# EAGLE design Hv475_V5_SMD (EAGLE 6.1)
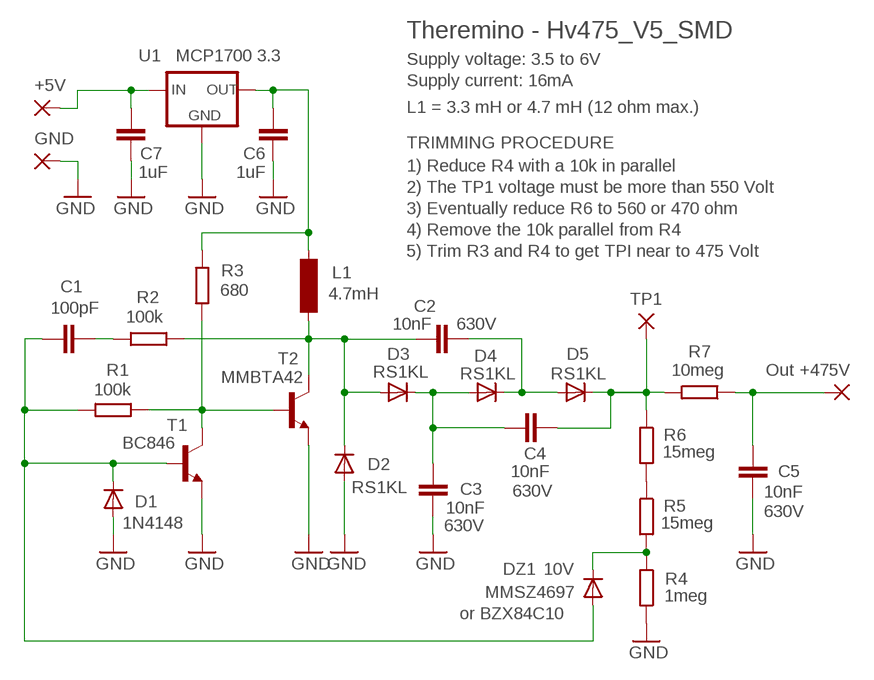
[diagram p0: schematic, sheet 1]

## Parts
+5V  WIREPADSMD2,54-3,81  [SMD2,54-3,81]
+475V  WIREPADSMD1,90-2,54  [SMD1,90-2,54]
C1  100pF  C-EUC0805  [C0805]
C2  10nF  C-EUC1206  [C1206]
C3  10nF  C-EUC1206  [C1206]
C4  10nF  C-EUC1206  [C1206]
C5  10nF  C-EUC1206  [C1206]
C6  1uF  C-EUC0805  [C0805]
C7  1uF  C-EUC0805  [C0805]
D1  1N4148  DIODE-SOD123-LARGE  [SOD123-LARGE]
D2  RS1KL  DIODE-SOD123-LARGE  [SOD123-LARGE]
D3  RS1KL  DIODE-SOD123-LARGE  [SOD123-LARGE]
D4  RS1KL  DIODE-SOD123-LARGE  [SOD123-LARGE]
D5  RS1KL  DIODE-SOD123-LARGE  [SOD123-LARGE]
DZ1  MMSZ4697  DIODE-SOD123-LARGE  [SOD123-LARGE]
GND  WIREPADSMD2,54-3,81  [SMD2,54-3,81]
L1  4.7mH  INDUCTOR_4.7MH472KU  [MSD75]
R1  100k  R-EU_R0805  [R0805]
R2  100k  R-EU_R0805  [R0805]
R3  680  R-EU_R1206_L  [R1206_L]
R4  1meg  R-EU_R0805  [R0805]
R5  15meg  R-EU_R1206  [R1206]
R6  15meg  R-EU_R1206  [R1206]
R7  10meg  R-EU_R1206  [R1206]
T1  BC846  BC846L  [SOT23_L@1]
T2  MMBTA42  -NPN-BC846  [SOT23_L@1]
TP1  TEST  WIREPADSMD1,27-1,27  [SMD1,27-1,27]
U1  MCP1700 3.3  MCP1700SOT23  [SOT23]

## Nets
+5V: C6.1 L1.1 R3.2 U1.2(OUT)
GND: C3.1 C5.1 C6.2 C7.2 D1.A D2.A GND.1(P) R4.1 T1.2(E) T2.2(E) U1.1(GND)
N$1: DZ1.C R4.2 R5.2
N$2: C1.2 R2.2
N$3: R5.1 R6.2
N$4: C1.1 D1.C DZ1.A R1.2 T1.1(B)
N$5: C4.2 D5.C R6.1 R7.2 TP1.1(P)
N$6: C2.1 D2.C D3.A L1.2 R2.1 T2.3(C)
N$7: +5V.1(P) C7.1 U1.3(IN)
N$11: C3.2 C4.1 D3.C D4.A
N$15: +475V.1(P) C5.2 R7.1
N$17: C2.2 D4.C D5.A
N$26: R1.1 R3.1 T1.3(C) T2.1(B)

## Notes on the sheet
- Theremino - Hv475_V5_SMD
- Supply voltage: 3.5 to 6V
- Supply current: 16mA
- L1 = 3.3 mH or 4.7 mH (12 ohm max.)
- TRIMMING PROCEDURE
- 1) Reduce R4 with a 10k in parallel
- 2) The TP1 voltage must be more than 550 Volt
- 3) Eventually reduce R6 to 560 or 470 ohm
- 4) Remove the 10k parallel from R4
- 5) Trim R3 and R4 to get TPI near to 475 Volt
- Out +475V

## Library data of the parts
+5V +475V GND TP1 = 00-LIVIO:WIREPAD: Wire PAD connect wire on PCB
C1 C6 C7 = 00-LIVIO:C-EU: CAPACITOR, European symbol
C2-C5 = 00-LIVIO:C-EU: CAPACITOR, European symbol; VOLTAGE: 630V
D1-D5 = 00-LIVIO:DIODE-: DIODE
DZ1 = 00-LIVIO:DIODE-: DIODE; EQUIVALENT: or BZX84C10; VZ: 10V
L1 = 00-LIVIO:INDUCTOR_4.7MH: INDUCTOR
R1-R7 = 00-LIVIO:R-EU_: RESISTOR, European symbol
T1 = 00-LIVIO:BC846
T2 = 00-LIVIO:*-NPN-: NPN Transistror
U1 = 00-LIVIO:MCP1700: Linear regulator Quescient courrent 1.8uA Input 2.3v to 6v Output 1.2v 1.8v 2.5v 3.0v 3.3v 5.0v

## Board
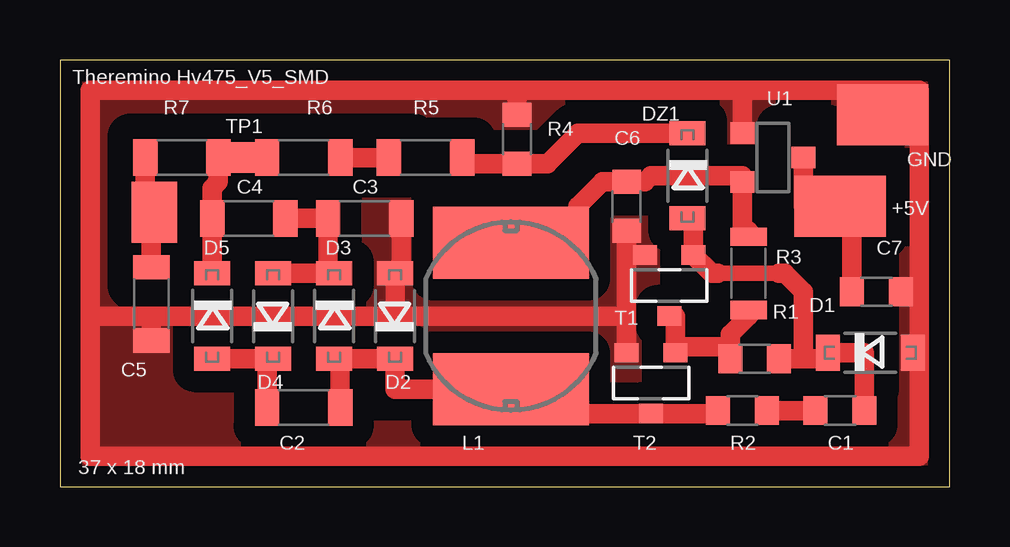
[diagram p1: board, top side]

Size 37.08 x 17.78 mm. Coordinates in mm from the lower left corner, seen from the top.
Outline: 0,0 37.08,0 37.08,17.78 0,17.78 0,0
Copper layers (1*16): Top 0.035mm / dielectric 1.5mm / Bottom 0.035mm
Design rules: minimum track width 10mil, minimum drill 0.6mm, track to track 8mil, track to pad 8mil, pad to pad 8mil, via to via 8mil, smd to smd 8mil, copper to edge 31mil, drill to drill 8mil, minimum pad ring 5mil, minimum via ring 8mil, stop-mask expansion 4mil, vias tented up to drill 0mil, thermal gap 47mil
tRestrict: 7 lines

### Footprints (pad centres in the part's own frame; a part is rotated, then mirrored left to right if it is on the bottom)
SMD2,54-3,81 = smd 2.54 x 3.81: 1 0,0
SMD1,90-2,54 = smd 1.905 x 2.54: 1 0,0
C0805 = smd 1 x 1.2: 1 -1.016,0; 2 1.016,0
C1206 = smd 1.016 x 1.524: 1 -1.524,0; 2 1.524,0
SOD123-LARGE = smd 1 x 1.5: A 1.778,0; C -1.778,0
MSD75 = smd 3 x 6.5: 1 3.048,0; 2 -3.048,0
R0805 = smd 1 x 1.2: 1 -1.016,0; 2 1.016,0
R1206_L = smd 0.762 x 1.524: 1 -1.524,0; 2 1.524,0
R1206 = smd 1.016 x 1.524: 1 -1.524,0; 2 1.524,0
SOT23_L@1 = smd 1 x 0.8: 1 -1.016,-1.27; 2 1.016,-1.27; 3 0,1.27
SMD1,27-1,27 = smd 1.27 x 1.27: 1 0,0
SOT23 = smd 0.889 x 1.016: 1 -1.016,-1.27; 2 1.016,-1.27; 3 0,1.27

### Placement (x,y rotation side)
+5V  32.51,11.68 90 top
+475V  3.94,11.43 0 top
C1  32.51,3.17 180 top
C2  10.16,3.3 180 top
C3  12.7,11.18 180 top
C4  7.87,11.18 180 top
C5  3.81,7.62 90 top
C6  23.62,11.68 270 top
C7  34.04,8.13 0 top
D1  33.78,5.59 0 top
D2  13.97,7.11 90 top
D3  11.43,7.11 270 top
D4  8.89,7.11 90 top
D5  6.35,7.11 270 top
DZ1  26.16,12.95 270 top
GND  34.29,15.49 90 top
L1  18.8,7.11 90 top
R1  28.96,5.33 0 top
R2  28.45,3.17 0 top
R3  28.7,8.89 90 top
R4  19.05,14.48 270 top
R5  15.24,13.72 0 top
R6  10.16,13.72 0 top
R7  5.08,13.72 0 top
T1  25.4,8.38 180 top
T2  24.64,4.32 180 top
TP1  7.62,13.72 180 top
U1  29.72,13.72 270 top

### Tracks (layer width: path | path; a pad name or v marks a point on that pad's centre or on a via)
+5V
  Top 0.7: R3.2 28.7,10.67
  Top 0.813: L1.1 18.8,10.92 21.59,10.92 21.59,11.68 22.61,12.7 C6.1 24.38,12.7 24.64,12.95 28.45,12.95 U1.2 28.45,10.67 28.7,10.67
GND
  Top 0.813: T2.2 23.62,7.11 | 23.62,7.11 13.97,7.11 | 13.97,7.11 3.81,7.11 | 3.81,7.11 1.27,7.11 | 13.97,7.11 D2.A 14.22,8.89 C3.1 | 35.81,5.59 35.81,1.27 1.27,1.27 1.27,7.11 | 35.81,5.59 35.81,8.13 | 35.81,8.13 35.81,16.51 34.29,16.51 | 34.29,16.51 28.45,16.51 | 28.45,16.51 19.05,16.51 | R4.1 19.05,16.51 | 19.05,16.51 1.27,16.51 1.27,7.11 | C5.1 3.81,7.11 | T1.2 23.62,9.65 | 23.62,9.65 23.62,7.11 | D1.A 35.81,5.59 | C6.2 23.62,9.65 | U1.1 28.45,16.51 | GND.1 34.29,16.51 | C7.2 35.81,8.13
  pour Top (isolate 0.9, rank 6, no thermals): -1,-1 38.08,-1 38.08,18.78 -1,18.78
N$1
  Top 0.813: R5.2 16.76,13.46 R4.2 20.32,13.46 21.59,14.73 DZ1.C
N$2
  Top 0.813: R2.2 C1.2
N$3
  Top 0.813: R5.1 R6.2
N$4
  Top 0.65: 27.43,8.89 29.97,8.89
  Top 0.813: C1.1 33.53,5.59 D1.C 32,5.33 30.99,5.33 | 27.43,8.89 27.18,8.89 T1.1 26.42,11.18 DZ1.A | 29.97,8.89 30.23,8.89 30.99,8.13 30.99,5.33 | R1.2 30.99,5.33
N$5
  Top 0.813: D5.C C4.2 6.35,12.45 6.6,12.7 R7.2 TP1.1 R6.1
N$6
  Top 0.813: C2.1 11.68,5.33 D3.A D2.C 13.97,4.06 L1.2 18.8,3.05 T2.3 27.43,3.05 R2.1
N$7
  Top 0.813: U1.3 30.99,11.68 +5V.1 33.02,11.68 C7.1
N$11
  Top 0.813: D4.A D3.C 11.18,8.89 C3.2 C4.1
N$15
  Top 0.813: C5.2 3.81,11.43 +475V.1 3.56,11.43 R7.1 3.56,13.97
N$17
  Top 0.813: D5.A D4.C 8.64,5.33 C2.2
N$26
  Top 0.7: 28.7,7.11 R3.1
  Top 0.813: T2.1 25.65,5.84 | 25.65,5.84 27.94,5.84 | 27.94,5.84 27.94,6.35 28.7,7.11 | R1.1 27.94,5.84 | T1.3 25.65,7.11 25.65,5.84

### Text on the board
tNames: Theremino Hv475_V5_SMD | 37 x 18 mm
